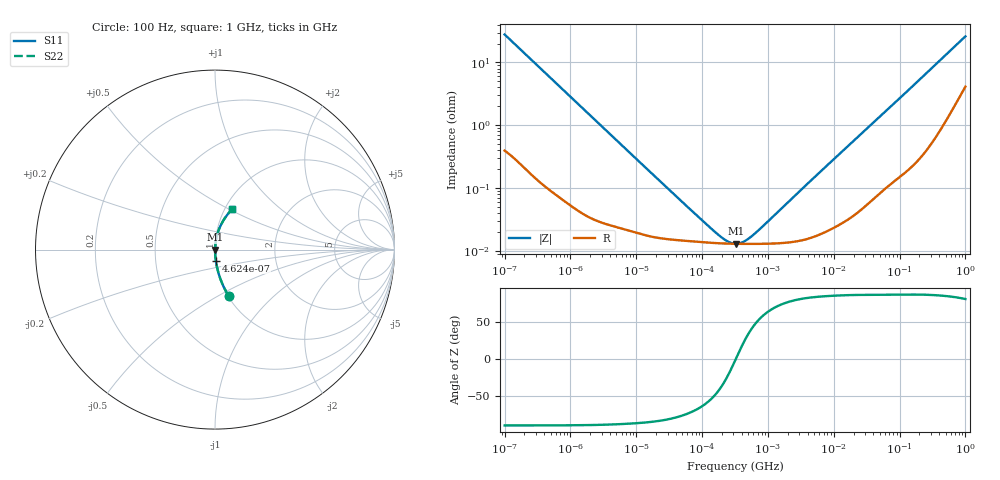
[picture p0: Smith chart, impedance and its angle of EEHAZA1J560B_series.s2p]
!  *** S-Parameter ***
!  Copyright (C) Panasonic Industry
!  Conductive Polymer Hybrid Aluminum Electrolytic Capacitor
!  Parts No. EEHAZA1J560B
!  Connection Mode : Series
!  1  o---||---o  2
!  GND o--------o GND
!  Conditions : Temperature = 20 degC , DC Bias = 0 V
! Frequency Range : 100Hz  -  1GHz  [ 401 Steps ]
# Hz S RI R 50
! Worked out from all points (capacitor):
!   401 points, 100 Hz to 1 GHz, reference 50 ohm
!   read as one part in series: C = 56.8 uF near 108.4 Hz
!   lowest |Z| = 13 mohm at 329.2 kHz (marker M1)
!   series resonance near 324.5 kHz, so ESL is about 4.2 nH
!   S11 on the Smith chart (normalised r, x): 100 Hz: 1.01, -0.56; 462.4 Hz: 1.00, -0.12; 1 GHz: 1.08, +0.51
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100  0.0754 -0.257  0.9246 0.257  0.9246 0.257  0.0754 -0.257
108.3927  0.0653 -0.24  0.9347 0.24  0.9347 0.24  0.0653 -0.24
206.538  0.0201 -0.1332  0.9799 0.1332  0.9799 0.1332  0.0201 -0.1332
296.8247  0.0103 -0.094  0.9897 0.094  0.9897 0.094  0.0103 -0.094
462.381  0.00469 -0.0609  0.9953 0.0609  0.9953 0.0609  0.00469 -0.0609
1487.647  0.000769 -0.0192  0.9992 0.0192  0.9992 0.0192  0.000769 -0.0192
22130.95  0.000163 -0.00133  0.9998 0.00133  0.9998 0.00133  0.000163 -0.00133
172782.6  0.000133 -0.000128  0.9999 0.000128  0.9999 0.000128  0.000133 -0.000128
238506.4  0.000131 -5.97e-05  0.9999 5.97e-05  0.9999 5.97e-05  0.000131 -5.97e-05
280220.6  0.000131 -2.82e-05  0.9999 2.82e-05  0.9999 2.82e-05  0.000131 -2.82e-05
316227.8  0.00013 -4.93e-06  0.9999 4.93e-06  0.9999 4.93e-06  0.00013 -4.93e-06
329230.5  0.00013 2.79e-06  0.9999 -2.79e-06  0.9999 -2.79e-06  0.00013 2.79e-06
371535.2  0.00013 2.61e-05  0.9999 -2.61e-05  0.9999 -2.61e-05  0.00013 2.61e-05
436515.8  0.00013 5.78e-05  0.9999 -5.78e-05  0.9999 -5.78e-05  0.00013 5.78e-05
602559.6  0.00013 0.000127  0.9999 -0.000127  0.9999 -0.000127  0.00013 0.000127
4704354  0.000166 0.00137  0.9998 -0.00137  0.9998 -0.00137  0.000166 0.00137
6.99842e7  0.00147 0.0189  0.9985 -0.0189  0.9985 -0.0189  0.00147 0.0189
1.566751e8  0.00395 0.0413  0.9961 -0.0413  0.9961 -0.0413  0.00395 0.0413
2.985383e8  0.011 0.0774  0.989 -0.0774  0.989 -0.0774  0.011 0.0774
5.688529e8  0.035 0.1415  0.965 -0.1415  0.965 -0.1415  0.035 0.1415
9.225714e8  0.0827 0.2109  0.9173 -0.2109  0.9173 -0.2109  0.0827 0.2109
1e9  0.0948 0.2235  0.9052 -0.2235  0.9052 -0.2235  0.0948 0.2235
